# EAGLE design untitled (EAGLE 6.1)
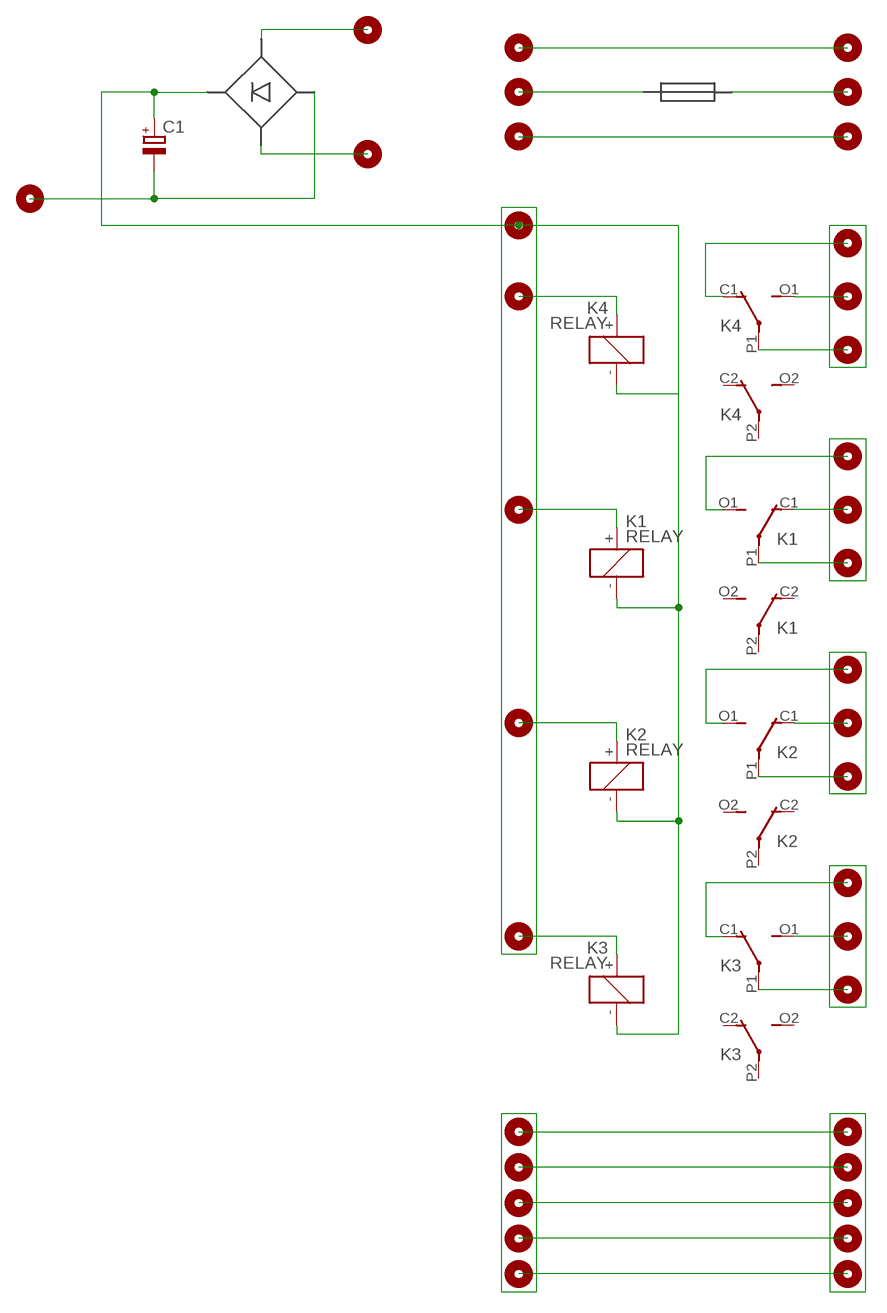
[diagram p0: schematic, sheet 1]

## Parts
C1  CPOL-EUE5-10.5  [E5-10,5]
K1  RELAY  [RELAY]
K2  RELAY  [RELAY]
K3  RELAY  [RELAY]
K4  RELAY  [RELAY]
U$1  PIN  [PIN]
U$2  PIN  [PIN]
U$3  PIN  [PIN]
U$4  PIN  [PIN]
U$5  PIN  [PIN]
U$6  PIN  [PIN]
U$7  PIN  [PIN]
U$8  PIN  [PIN]
U$9  PIN  [PIN]
U$10  PIN  [PIN]
U$11  PIN  [PIN]
U$12  PIN  [PIN]
U$13  PIN  [PIN]
U$14  PIN  [PIN]
U$15  PIN  [PIN]
U$16  PIN  [PIN]
U$17  PIN  [PIN]
U$18  PIN  [PIN]
U$19  PIN  [PIN]
U$20  PIN  [PIN]
U$21  PIN  [PIN]
U$22  PIN  [PIN]
U$23  PIN  [PIN]
U$24  PIN  [PIN]
U$25  PIN  [PIN]
U$26  PIN  [PIN]
U$27  PIN  [PIN]
U$28  PIN  [PIN]
U$29  PIN  [PIN]
U$30  PIN  [PIN]
U$31  FUE  [FUE]
U$32  DIODE  [DIODE]
U$33  PIN  [PIN]
U$34  PIN  [PIN]
U$35  PIN  [PIN]
U$36  PIN  [PIN]
U$37  PIN  [PIN]
U$39  PIN  [PIN]

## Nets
N$1: K4.P1(P) U$2.1
N$2: K4.O1(O) U$1.1
N$3: K4.C1(C) U$3.1
N$4: K1.O1(O) U$4.1
N$5: K1.C1(C) U$5.1
N$6: K1.P1(P) U$6.1
N$7: K2.O1(O) U$14.1
N$8: K2.C1(C) U$7.1
N$9: K2.P1(P) U$13.1
N$10: K3.O1(O) U$8.1
N$11: K3.C1(C) U$9.1
N$12: K3.P1(P) U$10.1
N$13: U$17.1 U$23.1
N$14: U$16.1 U$19.1
N$15: U$11.1 U$22.1
N$16: U$12.1 U$21.1
N$17: U$18.1 U$20.1
N$24: U$28.1 U$35.1
N$27: K4.+ U$25.1
N$28: K1.+ U$26.1
N$29: K2.+ U$27.1
N$30: K3.+ U$15.1
N$36: U$29.1 U$31.P$2 U$31.P$4
N$38: U$30.1 U$33.1
N$39: U$31.P$1 U$31.P$3 U$34.1
N$41: U$32.P U$36.1
N$45: U$32.P1 U$37.1
N$46: C1.+ K1.- K2.- K3.- K4.- U$24.1 U$32.+
N$47: C1.- U$32.- U$39.1
Unconnected: K1.C2(C) K1.O2(O) K1.P2(P) K2.C2(C) K2.O2(O) K2.P2(P) K3.C2(C) K3.O2(O) K3.P2(P) K4.C2(C) K4.O2(O) K4.P2(P)

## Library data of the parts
C1 = rcl:CPOL-EU: POLARIZED CAPACITOR, European symbol
K1-K4 = untitled:RELAY
U$1-U$30 U$33-U$37 U$39 = untitled:PIN
U$31 = untitled:FUE
U$32 = untitled:DIODE

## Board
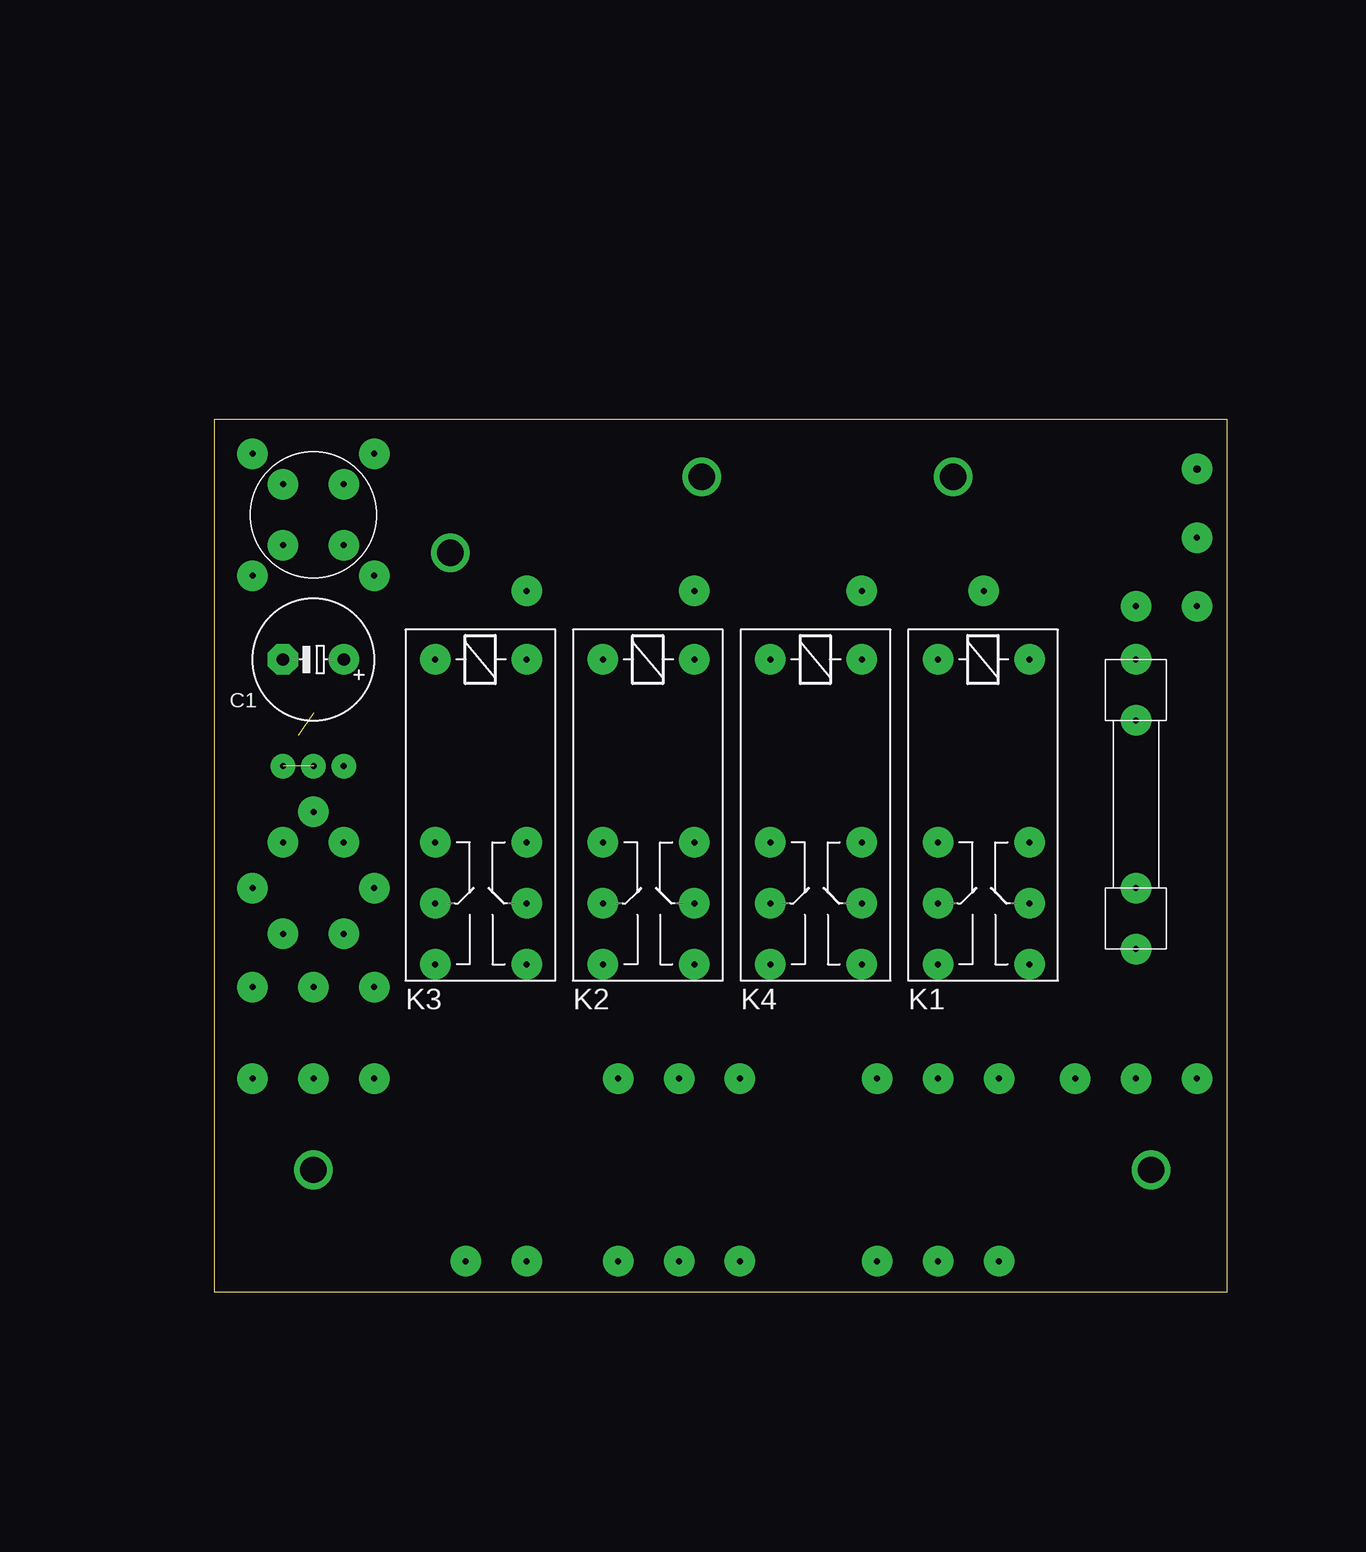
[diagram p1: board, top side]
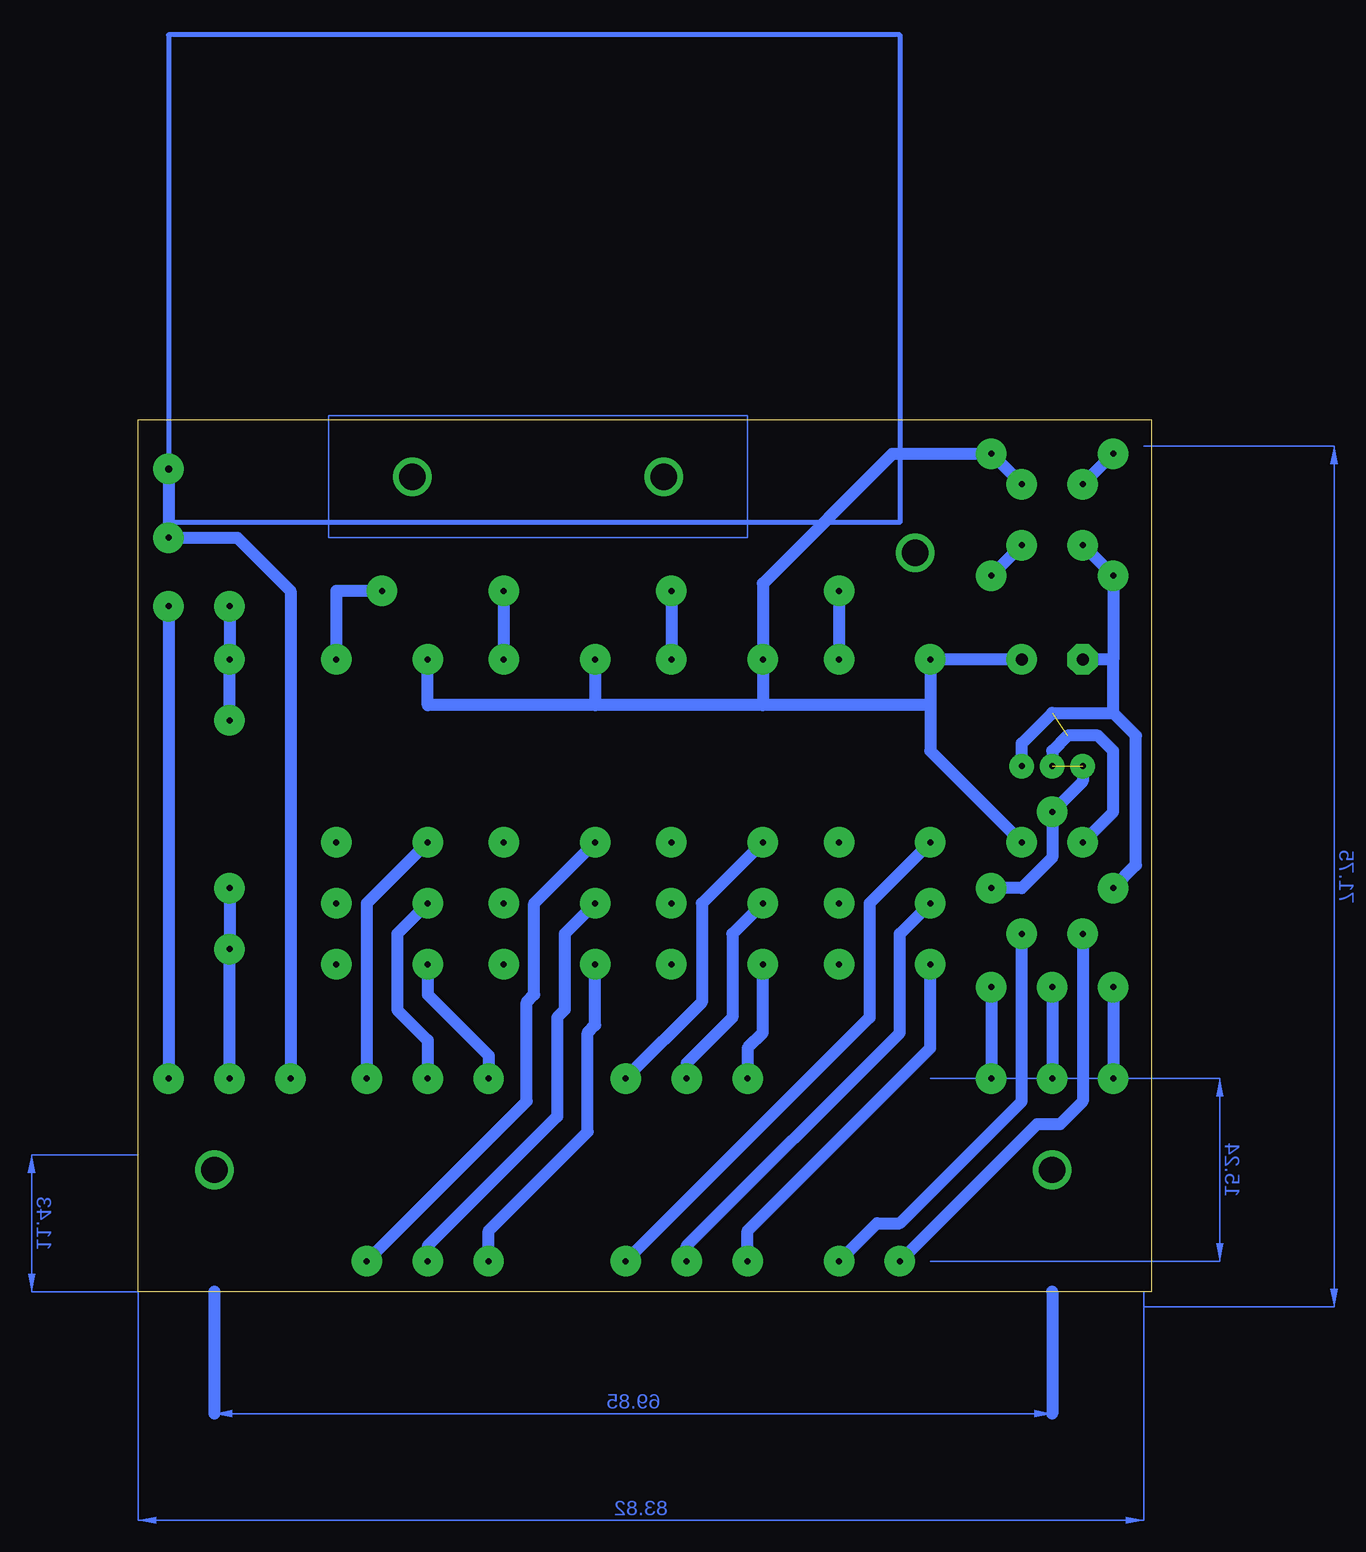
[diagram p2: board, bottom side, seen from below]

Size 84.44 x 72.69 mm. Coordinates in mm from the lower left corner, seen from the top.
Outline: 0,0 84.44,0 84.44,72.69 0,72.69 0,0
Copper layers (1*16): Top 0.035mm / dielectric 1.5mm / Bottom 0.035mm
Design rules: minimum track width 10mil, minimum drill 24mil, track to track 8mil, track to pad 8mil, pad to pad 8mil, via to via 8mil, smd to smd 8mil, copper to edge 40mil, drill to drill 8mil, minimum pad ring 10mil, minimum via ring 8mil, stop-mask expansion 4mil, vias tented up to drill 0mil, thermal gap 10mil

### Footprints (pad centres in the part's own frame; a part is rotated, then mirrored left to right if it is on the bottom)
E5-10,5 = drill 1.016 pad 2.54: + -2.54,0 | drill 1.016 pad 2.54 octagon: - 2.54,0
RELAY = drill 0.5 pad 2.54: + -10.795,3.81; - -10.795,-3.81; C1 4.445,-3.81; C2 4.445,3.81; O1 14.605,-3.81; O2 14.605,3.81; P1 9.525,-3.81; P2 9.525,3.81
PIN = drill 0.5 pad 1.676 square: 1 0,0
FUE = drill 0.5 pad 2.54: P$1 16.51,0; P$2 2.54,0; P$3 21.59,0; P$4 -2.54,0
DIODE = drill 0.5 pad 2.54: + -3.81,-5.08; - 1.27,0; P -3.81,0; P1 1.27,-5.08

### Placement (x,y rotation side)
C1  8.26,52.7 180 top
K1  64.14,41.91 270 top
K2  36.2,41.91 270 top
K3  22.23,41.91 270 top
K4  50.16,41.91 270 top
U$1  55.24,2.54 0 top
U$2  60.32,2.54 0 top
U$3  65.41,2.54 0 top
U$4  55.24,17.78 0 top
U$5  65.41,17.78 0 top
U$6  60.32,17.78 0 top
U$7  43.81,17.78 0 top
U$8  33.66,2.54 0 top
U$9  43.81,2.54 0 top
U$10  38.73,2.54 0 top
U$11  20.96,2.54 0 top
U$12  26.04,2.54 0 top
U$13  38.73,17.78 0 top
U$14  33.66,17.78 0 top
U$15  26.04,58.42 0 top
U$16  13.33,17.78 0 top
U$17  8.26,17.78 0 top
U$18  3.17,17.78 0 top
U$19  13.33,25.4 0 top
U$20  3.17,25.4 0 top
U$21  10.79,29.84 0 top
U$22  5.71,29.84 0 top
U$23  8.26,25.4 0 top
U$24  13.33,69.85 0 top
U$25  53.98,58.42 0 top
U$26  64.14,58.42 0 top
U$27  40,58.42 0 top
U$28  71.76,17.78 0 top
U$29  76.84,17.78 0 top
U$30  81.92,17.78 0 top
U$31  76.84,31.11 90 top
U$32  6.98,62.23 180 top
U$33  81.92,57.15 0 top
U$34  76.84,57.15 0 top
U$35  81.92,62.87 0 top
U$36  13.33,59.69 0 top
U$37  3.17,69.85 0 top
U$39  3.17,59.69 0 top

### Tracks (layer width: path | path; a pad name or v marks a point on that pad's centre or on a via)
N$1  (via drill 0.5 pad 2.54)
  Bottom 1.016: U$2.1 60.32,3.81 49.53,14.61 49.53,22.86 48.89,23.5 48.89,29.84 K4.P1
  other vias: 60.32,2.54
N$2
  Bottom 1.016: U$1.1 55.24,5.08 46.99,13.34 46.99,21.59 46.35,22.23 K4.O1
N$3
  Bottom 1.016: U$3.1 52.07,15.88 52.07,24.13 51.43,24.77 51.43,32.38 K4.C1
N$4
  Bottom 1.016: U$4.1 55.24,19.68 60.32,24.77 K1.O1
N$5
  Bottom 1.016: U$5.1 65.41,32.38 K1.C1
N$6
  Bottom 1.016: U$6.1 60.32,20.95 62.86,23.5 62.86,29.84 K1.P1
N$7
  Bottom 1.016: U$14.1 33.66,20.32 32.38,21.59 K2.O1
N$8
  Bottom 1.016: U$7.1 37.46,24.13 37.46,32.38 K2.C1
N$9
  Bottom 1.016: U$13.1 38.73,19.05 34.92,22.86 34.92,29.84 K2.P1
N$10
  Bottom 1.016: U$8.1 33.66,5.08 18.42,20.32 K3.O1
N$11
  Bottom 1.016: K3.C1 23.5,32.38 23.5,22.86 U$9.1
N$12
  Bottom 1.016: U$10.1 38.73,3.81 20.96,21.59 20.96,29.84 K3.P1
N$13
  Bottom 1.016: U$23.1 U$17.1
N$14
  Bottom 1.016: U$19.1 U$16.1
N$15
  Bottom 1.016: U$22.1 5.71,15.88 7.62,13.97 9.53,13.97 U$11.1
N$16
  Bottom 1.016: U$12.1 22.86,5.71 20.96,5.71 10.79,15.88 U$21.1
N$17
  Bottom 1.016: U$20.1 U$18.1
N$18  (via drill 2.2 pad 2.18)
  other vias: 78.11,10.16
N$19
  Bottom 0.127: 33.66,62.87 68.58,62.87 68.58,73.03 33.66,73.03 33.66,62.87
N$20
  Bottom 1.016: 78.11,0 78.11,-10.16
N$21
  Bottom 1.016: 8.26,0 8.26,-10.16
N$22  (via drill 2.2 pad 2.18)
  other vias: 40.64,67.94
N$23  (via drill 2.2 pad 2.18)
  other vias: 61.59,67.94
N$24  (via drill 0.6 pad 1.68)
  Bottom 1.016: U$28.1 71.76,58.42 76.2,62.87 U$35.1 v81.92,68.58
N$25  (via drill 2.2 pad 2.18)
  other vias: 8.26,10.16
N$26  (via drill 2.2 pad 2.18)
  other vias: 19.69,61.59
N$27
  Bottom 1.016: U$25.1 K4.+
N$28
  Bottom 1.016: U$26.1 67.95,58.42 K1.+
N$29
  Bottom 1.016: U$27.1 K2.+
N$30
  Bottom 1.016: U$15.1 K3.+
N$35
  Bottom 0.406: 20.96,64.14 81.92,64.14 81.92,104.78 20.96,104.78 20.96,64.14
N$36
  Bottom 1.016: U$29.1 U$31.P$4 U$31.P$2
N$38
  Bottom 1.016: U$33.1 U$30.1
N$39
  Bottom 1.016: U$34.1 U$31.P$3 U$31.P$1
N$41
  Bottom 1.016: U$32.P U$36.1
N$45
  Bottom 1.016: U$37.1 U$32.P1
N$46  (via drill 0.5 pad 2.54)
  Bottom 1.016: 18.42,48.9 K3.- C1.+ | 18.42,48.9 32.38,48.9 | 32.38,48.9 46.35,48.9 | 46.35,48.9 60.32,48.9 K1.- | K4.- 46.35,48.9 | 32.38,48.9 K2.- 32.38,59.05 21.59,69.85 U$24.1 U$32.+ | 18.42,48.9 18.42,45.09 v10.79,37.47
N$47  (via drill 0.5 pad 2.03, 0.5 pad 2.54)  (2 unrouted)
  Bottom 1.016: U$32.- U$39.1 3.17,52.7 | 3.17,52.7 C1.- | v3.17,33.66 1.27,35.56 1.27,46.35 3.17,48.26 | 3.17,48.26 3.17,52.7 | v5.71,37.47 3.17,40.01 3.17,45.09 4.45,46.35 6.98,46.35 8.26,45.09 v8.26,43.81 | v5.71,43.81 5.71,42.55 v8.26,40.01 8.26,36.2 10.79,33.66 v13.33,33.66 | v10.79,43.81 10.79,45.72 8.26,48.26 3.17,48.26
S$1  (via drill 0.5 pad 2.54)
  other vias: 5.71,29.84
S$2  (via drill 0.5 pad 2.54)
  other vias: 10.79,29.84
S$3  (via drill 0.5 pad 2.54)
  other vias: 13.33,25.4
S$4  (via drill 0.5 pad 2.54)
  other vias: 8.26,25.4
S$5  (via drill 0.5 pad 2.54)
  other vias: 3.17,25.4
S$6  (via drill 0.5 pad 2.54)
  other vias: 13.33,59.69
S$7  (via drill 0.5 pad 2.54)
  other vias: 3.17,59.69
S$8  (via drill 0.5 pad 2.54)
  other vias: 26.04,58.42
S$9  (via drill 0.5 pad 2.54)
  other vias: 40,58.42
S$10  (via drill 0.5 pad 2.54)
  other vias: 53.98,58.42
S$11  (via drill 0.5 pad 2.54)
  other vias: 64.14,58.42
S$13  (via drill 0.5 pad 2.54)
  other vias: 3.17,69.85 13.33,69.85
S$14  (via drill 0.5 pad 2.54)
  other vias: 81.92,57.15
S$15  (via drill 0.5 pad 2.54)
  other vias: 76.84,57.15
S$16  (via drill 0.5 pad 2.54)
  other vias: 81.92,62.87
S$17  (via drill 0.5 pad 2.54)
  other vias: 81.92,68.58
S$18  (via drill 0.5 pad 2.54)
  other vias: 81.92,17.78
S$19  (via drill 0.5 pad 2.54)
  other vias: 76.84,17.78
S$20  (via drill 0.5 pad 2.54)
  other vias: 71.76,17.78
S$21  (via drill 0.5 pad 2.54)
  other vias: 65.41,17.78
S$22  (via drill 0.5 pad 2.54)
  other vias: 60.32,17.78
S$23  (via drill 0.5 pad 2.54)
  other vias: 55.24,17.78
S$24  (via drill 0.5 pad 2.54)
  other vias: 43.81,17.78
S$25  (via drill 0.5 pad 2.54)
  other vias: 38.73,17.78
S$26  (via drill 0.5 pad 2.54)
  other vias: 33.66,17.78
S$27  (via drill 0.5 pad 2.54)
  other vias: 13.33,17.78
S$28  (via drill 0.5 pad 2.54)
  other vias: 8.26,17.78
S$29  (via drill 0.5 pad 2.54)
  other vias: 3.17,17.78
S$30  (via drill 0.5 pad 2.54)
  other vias: 65.41,2.54
S$31  (via drill 0.5 pad 2.54)
  other vias: 55.24,2.54
S$32  (via drill 0.5 pad 2.54)
  other vias: 38.73,2.54
S$33  (via drill 0.5 pad 2.54)
  other vias: 33.66,2.54
S$34  (via drill 0.5 pad 2.54)
  other vias: 43.81,2.54
S$35  (via drill 0.5 pad 2.54)
  other vias: 26.04,2.54
S$36  (via drill 0.5 pad 2.54)
  other vias: 20.96,2.54
(copper drawn outside any net)
  shapes: Bottom area x5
